| Teraspeed Modeling Services.
| http://www.teraspeed.com
[IBIS Ver]   4.0
[Comment Char] |_char
[File Name]   lpc812m101fdh20_ht.ibs
[File Rev]   3.0
[Source]  Measured and created by Teraspeed Consulting Group LLC
[Date]   08-09-2013
[Notes]   Quality Check of this IBIS model: Model Passes IBIS Check
   Model parses into ICX IS. Simulation done with Hyperlynx.
   1. MIN TYP MAX information is based on Temperature and Voltage
   characteristics only.
   2. Package data measured using Tektronix IConnect Software.
   3. This model higher temperature range:  -40 to +105
[Disclaimer]
| Use: Teraspeed Consulting Group LLC ("Teraspeed") has
| licensed IBIS models to specific integrated circuit
| suppliers ("IC Vendors") for use and distribustion as
| follows: Each IC Vendor may use IBIS Models, and distribute
| them to IC Vendor's custumers to use solely for developing
| printed circute board designs. Users of this model may
| modify the IBIS model to suit its specific applications but
| rights to derivative works and such modifications shall belong
| to Teraspeed. No other distribution of these materials is
| permitted.
| DISCLAIMER OF WARRANTY: UNLESS OTHERWISE AGREED TO IN WRITING
| TERASPEED DISCLAIMS AND USER WAIVES ALL WARRANTIES, EXPRESS
| OR IMPLIED, INCLUDING WARRANTIES OF MERCHANTABILITY AND
| FITNESS FOR A PARTICULAR PURPOSE. IN NO EVENT SHALL
| TERASPEED BE LIABLE FOR ANY DIRECT OR INDIRECT DAMAGES,
| WHETHER IN CONTRACT OR TORT, INCLUDING, WITHOUT LIMITATION,
| LOST PROFITS, BUSINESS INTERRUPTION, OR LOST INFORMATION
| ARISING OUT OF THE USE OF OR THE INABILITY TO USE THE MODEL,
| EVEN IF TERASPEED HAS BEEN ADVISED OF THE POSSIBILITY OF SUCH
| DAMAGES.
[Copyright]
| This file is the legal property of Teraspeed Copyright(c) 2013.
| All other rights are reserved.
[Component] LPC812M101FDH20_HT
[Manufacturer] NXP Semiconductors
[Package]
| TSSOP20/SOT360-1
| variable   typ   min   max
R_pkg  1.000E-02  1.000E-02  1.000E-02
L_pkg  2.930E-09  2.280E-09  3.580E-09
C_pkg  8.810E-13  8.040E-13  9.580E-13
[Pin] signal_name  model_name  R_pin  L_pin C_pin
1   PIO0_17   pio0_17   1.000E-02   2.280E-09   8.040E-13
2   PIO0_13   pio0_13   1.000E-02   2.605E-09   8.425E-13
3   PIO0_12   pio0_12   1.000E-02   2.930E-09   8.810E-13
4   *RESET/PIO0_5   pio0_5   1.000E-02   3.255E-09   9.195E-13
5   PIO0_4/WAKEUP/*TRST   pio0_4   1.000E-02   3.580E-09   9.580E-13
6   SWCLK/PIO0_3/TCK   pio0_3   1.000E-02   3.580E-09   9.580E-13
7   SWDIO/PIO0_2/TMS   pio0_2   1.000E-02   3.255E-09   9.195E-13
8   PIO0_11   pio0_11   1.000E-02   2.930E-09   8.810E-13
9   PIO0_10   pio0_10   1.000E-02   2.605E-09   8.425E-13
10   PIO0_16   pio0_16   1.000E-02   2.280E-09   8.040E-13
11   PIO0_15   pio0_15   1.000E-02   2.280E-09   8.040E-13
12   PIO0_1/CMPI2/CLK/TDI   pio0_1   1.000E-02   2.605E-09   8.425E-13
13   PIO0_9/XTALOUT   pio0_9   1.000E-02   2.930E-09   8.810E-13
14   PIO0_8/XTALIN   pio0_8   1.000E-02   3.255E-09   9.195E-13
15   VDD   POWER   1.000E-02   3.580E-09   9.580E-13
16   VSS   GND   1.000E-02   3.580E-09   9.580E-13
17   PIO0_7   pio0_7   1.000E-02   3.255E-09   9.195E-13
18   PIO0_6/VDDCMP   pio0_6   1.000E-02   2.930E-09   8.810E-13
19   PIO0_0/CMPI1/TDO   pio0_0   1.000E-02   2.605E-09   8.425E-13
20   PIO0_14   pio0_14   1.000E-02   2.280E-09   8.040E-13
|******Normal Drive I/O's******
[Model Selector]  pio0_4
input_1.8v   input,no int pd/pu,vdd=1.8v
input_2.5v   input,no int pd/pu,vdd=2.5v
input_3.3v   input,no int pd/pu,vdd=3.3v
pd_1.8v   input,int pd,vdd=1.8v
pd_2.5v   input,int pd,vdd=2.5v
pd_3.3v   input,int pd,vdd=3.3v
pu_1.8v   input,int pu,vdd=1.8v | PWR-UP Default
pu_2.5v   input,int pu,vdd=2.5v | PWR-UP Default
pu_3.3v   input,int pu,vdd=3.3v | PWR-UP Default
io_1.8v   io,vdd=1.8v
io_2.5v   io,vdd=2.5v
io_3.3v   io,vdd=3.3v
io_odf_1.8v   fast open drain io,vdd=1.8v
io_odf_2.5v   fast open drain io,vdd=2.5v
io_odf_3.3v   fast open drain io,vdd=3.3v
[Model Selector]  pio0_5
input_1.8v   input,no int pd/pu,vdd=1.8v
input_2.5v   input,no int pd/pu,vdd=2.5v
input_3.3v   input,no int pd/pu,vdd=3.3v
pd_1.8v   input,int pd,vdd=1.8v
pd_2.5v   input,int pd,vdd=2.5v
pd_3.3v   input,int pd,vdd=3.3v
pu_1.8v   input,int pu,vdd=1.8v | PWR-UP/Reset Default
pu_2.5v   input,int pu,vdd=2.5v | PWR-UP/Reset Default
pu_3.3v   input,int pu,vdd=3.3v | PWR-UP/Reset Default
io_1.8v   io,vdd=1.8v
io_2.5v   io,vdd=2.5v
io_3.3v   io,vdd=3.3v
io_odf_1.8v   fast open drain io,vdd=1.8v
io_odf_2.5v   fast open drain io,vdd=2.5v
io_odf_3.3v   fast open drain io,vdd=3.3v
[Model Selector]  pio0_6
input_1.8v   input,no int pd/pu,vdd=1.8v
input_2.5v   input,no int pd/pu,vdd=2.5v
input_3.3v   input,no int pd/pu,vdd=3.3v
pd_1.8v   input,int pd,vdd=1.8v
pd_2.5v   input,int pd,vdd=2.5v
pd_3.3v   input,int pd,vdd=3.3v
pu_1.8v   input,int pu,vdd=1.8v | PWR-UP/Reset Default
pu_2.5v   input,int pu,vdd=2.5v | PWR-UP/Reset Default
pu_3.3v   input,int pu,vdd=3.3v | PWR-UP/Reset Default
io_1.8v   io,vdd=1.8v
io_2.5v   io,vdd=2.5v
io_3.3v   io,vdd=3.3v
io_odf_1.8v   fast open drain io,vdd=1.8v
io_odf_2.5v   fast open drain io,vdd=2.5v
io_odf_3.3v   fast open drain io,vdd=3.3v
[Model Selector]  pio0_14
input_1.8v   input,no int pd/pu,vdd=1.8v
input_2.5v   input,no int pd/pu,vdd=2.5v
input_3.3v   input,no int pd/pu,vdd=3.3v
pd_1.8v   input,int pd,vdd=1.8v
pd_2.5v   input,int pd,vdd=2.5v
pd_3.3v   input,int pd,vdd=3.3v
pu_1.8v   input,int pu,vdd=1.8v | PWR-UP/Reset Default
pu_2.5v   input,int pu,vdd=2.5v | PWR-UP/Reset Default
pu_3.3v   input,int pu,vdd=3.3v | PWR-UP/Reset Default
io_1.8v   io,vdd=1.8v
io_2.5v   io,vdd=2.5v
io_3.3v   io,vdd=3.3v
io_odf_1.8v   fast open drain io,vdd=1.8v
io_odf_2.5v   fast open drain io,vdd=2.5v
io_odf_3.3v   fast open drain io,vdd=3.3v
[Model Selector]  pio0_15
input_1.8v   input,no int pd/pu,vdd=1.8v
input_2.5v   input,no int pd/pu,vdd=2.5v
input_3.3v   input,no int pd/pu,vdd=3.3v
pd_1.8v   input,int pd,vdd=1.8v
pd_2.5v   input,int pd,vdd=2.5v
pd_3.3v   input,int pd,vdd=3.3v
pu_1.8v   input,int pu,vdd=1.8v | PWR-UP/Reset Default
pu_2.5v   input,int pu,vdd=2.5v | PWR-UP/Reset Default
pu_3.3v   input,int pu,vdd=3.3v | PWR-UP/Reset Default
io_1.8v   io,vdd=1.8v
io_2.5v   io,vdd=2.5v
io_3.3v   io,vdd=3.3v
io_odf_1.8v   fast open drain io,vdd=1.8v
io_odf_2.5v   fast open drain io,vdd=2.5v
io_odf_3.3v   fast open drain io,vdd=3.3v
[Model Selector]  pio0_16
input_1.8v   input,no int pd/pu,vdd=1.8v
input_2.5v   input,no int pd/pu,vdd=2.5v
input_3.3v   input,no int pd/pu,vdd=3.3v
pd_1.8v   input,int pd,vdd=1.8v
pd_2.5v   input,int pd,vdd=2.5v
pd_3.3v   input,int pd,vdd=3.3v
pu_1.8v   input,int pu,vdd=1.8v | PWR-UP/Reset Default
pu_2.5v   input,int pu,vdd=2.5v | PWR-UP/Reset Default
pu_3.3v   input,int pu,vdd=3.3v | PWR-UP/Reset Default
io_1.8v   io,vdd=1.8v
io_2.5v   io,vdd=2.5v
io_3.3v   io,vdd=3.3v
io_odf_1.8v   fast open drain io,vdd=1.8v
io_odf_2.5v   fast open drain io,vdd=2.5v
io_odf_3.3v   fast open drain io,vdd=3.3v
[Model Selector]  pio0_17
input_1.8v   input,no int pd/pu,vdd=1.8v
input_2.5v   input,no int pd/pu,vdd=2.5v
input_3.3v   input,no int pd/pu,vdd=3.3v
pd_1.8v   input,int pd,vdd=1.8v
pd_2.5v   input,int pd,vdd=2.5v
pd_3.3v   input,int pd,vdd=3.3v
pu_1.8v   input,int pu,vdd=1.8v | PWR-UP/Reset Default
pu_2.5v   input,int pu,vdd=2.5v | PWR-UP/Reset Default
pu_3.3v   input,int pu,vdd=3.3v | PWR-UP/Reset Default
io_1.8v   io,vdd=1.8v
io_2.5v   io,vdd=2.5v
io_3.3v   io,vdd=3.3v
io_odf_1.8v   fast open drain io,vdd=1.8v
io_odf_2.5v   fast open drain io,vdd=2.5v
io_odf_3.3v   fast open drain io,vdd=3.3v
|******Normal Drive I/O's w/Analog Func ******
[Model Selector]  pio0_0
input_1.8v   input,no int pd/pu,vdd=1.8v
input_2.5v   input,no int pd/pu,vdd=2.5v
input_3.3v   input,no int pd/pu,vdd=3.3v
pd_1.8v   input,int pd,vdd=1.8v
pd_2.5v   input,int pd,vdd=2.5v
pd_3.3v   input,int pd,vdd=3.3v
pu_1.8v   input,int pu,vdd=1.8v | PWR-UP/Reset Default
pu_2.5v   input,int pu,vdd=2.5v | PWR-UP/Reset Default
pu_3.3v   input,int pu,vdd=3.3v | PWR-UP/Reset Default
io_1.8v   io,vdd=1.8v
io_2.5v   io,vdd=2.5v
io_3.3v   io,vdd=3.3v
io_odf_1.8v   fast open drain io,vdd=1.8v
io_odf_2.5v   fast open drain io,vdd=2.5v
io_odf_3.3v   fast open drain io,vdd=3.3v
term   analog comparator input1
[Model Selector]  pio0_1
input_1.8v   input,no int pd/pu,vdd=1.8v
input_2.5v   input,no int pd/pu,vdd=2.5v
input_3.3v   input,no int pd/pu,vdd=3.3v
pd_1.8v   input,int pd,vdd=1.8v
pd_2.5v   input,int pd,vdd=2.5v
pd_3.3v   input,int pd,vdd=3.3v
pu_1.8v   input,int pu,vdd=1.8v | PWR-UP/Reset Default
pu_2.5v   input,int pu,vdd=2.5v | PWR-UP/Reset Default
pu_3.3v   input,int pu,vdd=3.3v | PWR-UP/Reset Default
io_1.8v   io,vdd=1.8v
io_2.5v   io,vdd=2.5v
io_3.3v   io,vdd=3.3v
io_odf_1.8v   fast open drain io,vdd=1.8v
io_odf_2.5v   fast open drain io,vdd=2.5v
io_odf_3.3v   fast open drain io,vdd=3.3v
term   analog comparator input2
[Model Selector]  pio0_8
input_1.8v   input,no int pd/pu,vdd=1.8v
input_2.5v   input,no int pd/pu,vdd=2.5v
input_3.3v   input,no int pd/pu,vdd=3.3v
pd_1.8v   input,int pd,vdd=1.8v
pd_2.5v   input,int pd,vdd=2.5v
pd_3.3v   input,int pd,vdd=3.3v
pu_1.8v   input,int pu,vdd=1.8v | PWR-UP/Reset Default
pu_2.5v   input,int pu,vdd=2.5v | PWR-UP/Reset Default
pu_3.3v   input,int pu,vdd=3.3v | PWR-UP/Reset Default
io_1.8v   io,vdd=1.8v
io_2.5v   io,vdd=2.5v
io_3.3v   io,vdd=3.3v
io_odf_1.8v   fast open drain io,vdd=1.8v
io_odf_2.5v   fast open drain io,vdd=2.5v
io_odf_3.3v   fast open drain io,vdd=3.3v
term   analog xtal in
[Model Selector]  pio0_9
input_1.8v   input,no int pd/pu,vdd=1.8v
input_2.5v   input,no int pd/pu,vdd=2.5v
input_3.3v   input,no int pd/pu,vdd=3.3v
pd_1.8v   input,int pd,vdd=1.8v
pd_2.5v   input,int pd,vdd=2.5v
pd_3.3v   input,int pd,vdd=3.3v
pu_1.8v   input,int pu,vdd=1.8v | PWR-UP/Reset Default
pu_2.5v   input,int pu,vdd=2.5v | PWR-UP/Reset Default
pu_3.3v   input,int pu,vdd=3.3v | PWR-UP/Reset Default
io_1.8v   io,vdd=1.8v
io_2.5v   io,vdd=2.5v
io_3.3v   io,vdd=3.3v
io_odf_1.8v   fast open drain io,vdd=1.8v
io_odf_2.5v   fast open drain io,vdd=2.5v
io_odf_3.3v   fast open drain io,vdd=3.3v
term   analog xtal out
|******High Drive(source) I/O's******
[Model Selector]  pio0_2
input_1.8v   input,no int pd/pu,vdd=1.8v
input_2.5v   input,no int pd/pu,vdd=2.5v
input_3.3v   input,no int pd/pu,vdd=3.3v
pd_1.8v   input,int pd,vdd=1.8v
pd_2.5v   input,int pd,vdd=2.5v
pd_3.3v   input,int pd,vdd=3.3v
pu_1.8v   input,int pu,vdd=1.8v | PWR-UP/Reset Default
pu_2.5v   input,int pu,vdd=2.5v | PWR-UP/Reset Default
pu_3.3v   input,int pu,vdd=3.3v | PWR-UP/Reset Default
hi_drv_io_1.8v  io,hi src drv,vdd=1.8v
hi_drv_io_2.5v  io,hi src drv,vdd=2.5v
hi_drv_io_3.3v  io,hi src drv,vdd=3.3v
io_ods_1.8v   slow open drain io,vdd=1.8v
io_ods_2.5v   slow open drain io,vdd=2.5v
io_ods_3.3v   slow open drain io,vdd=3.3v
[Model Selector]  pio0_3
input_1.8v   input,no int pd/pu,vdd=1.8v
input_2.5v   input,no int pd/pu,vdd=2.5v
input_3.3v   input,no int pd/pu,vdd=3.3v
pd_1.8v   input,int pd,vdd=1.8v
pd_2.5v   input,int pd,vdd=2.5v
pd_3.3v   input,int pd,vdd=3.3v
pu_1.8v   input,int pu,vdd=1.8v | PWR-UP/Reset Default
pu_2.5v   input,int pu,vdd=2.5v | PWR-UP/Reset Default
pu_3.3v   input,int pu,vdd=3.3v | PWR-UP/Reset Default
hi_drv_io_1.8v  io,hi src drv,vdd=1.8v
hi_drv_io_2.5v  io,hi src drv,vdd=2.5v
hi_drv_io_3.3v  io,hi src drv,vdd=3.3v
io_ods_1.8v   slow open drain io,vdd=1.8v
io_ods_2.5v   slow open drain io,vdd=2.5v
io_ods_3.3v   slow open drain io,vdd=3.3v
[Model Selector]  pio0_7
input_1.8v   input,no int pd/pu,vdd=1.8v
input_2.5v   input,no int pd/pu,vdd=2.5v
input_3.3v   input,no int pd/pu,vdd=3.3v
pd_1.8v   input,int pd,vdd=1.8v
pd_2.5v   input,int pd,vdd=2.5v
pd_3.3v   input,int pd,vdd=3.3v
pu_1.8v   input,int pu,vdd=1.8v | PWR-UP/Reset Default
pu_2.5v   input,int pu,vdd=2.5v | PWR-UP/Reset Default
pu_3.3v   input,int pu,vdd=3.3v | PWR-UP/Reset Default
hi_drv_io_1.8v  io,hi src drv,vdd=1.8v
hi_drv_io_2.5v  io,hi src drv,vdd=2.5v
hi_drv_io_3.3v  io,hi src drv,vdd=3.3v
io_ods_1.8v   slow open drain io,vdd=1.8v
io_ods_2.5v   slow open drain io,vdd=2.5v
io_ods_3.3v   slow open drain io,vdd=3.3v
[Model Selector]  pio0_12
input_1.8v   input,no int pd/pu,vdd=1.8v
input_2.5v   input,no int pd/pu,vdd=2.5v
input_3.3v   input,no int pd/pu,vdd=3.3v
pd_1.8v   input,int pd,vdd=1.8v
pd_2.5v   input,int pd,vdd=2.5v
pd_3.3v   input,int pd,vdd=3.3v
pu_1.8v   input,int pu,vdd=1.8v | PWR-UP/Reset Default
pu_2.5v   input,int pu,vdd=2.5v | PWR-UP/Reset Default
pu_3.3v   input,int pu,vdd=3.3v | PWR-UP/Reset Default
hi_drv_io_1.8v  io,hi src drv,vdd=1.8v
hi_drv_io_2.5v  io,hi src drv,vdd=2.5v
hi_drv_io_3.3v  io,hi src drv,vdd=3.3v
io_ods_1.8v   slow open drain io,vdd=1.8v
io_ods_2.5v   slow open drain io,vdd=2.5v
io_ods_3.3v   slow open drain io,vdd=3.3v
[Model Selector]  pio0_13
input_1.8v   input,no int pd/pu,vdd=1.8v
input_2.5v   input,no int pd/pu,vdd=2.5v
input_3.3v   input,no int pd/pu,vdd=3.3v
pd_1.8v   input,int pd,vdd=1.8v
pd_2.5v   input,int pd,vdd=2.5v
pd_3.3v   input,int pd,vdd=3.3v
pu_1.8v   input,int pu,vdd=1.8v | PWR-UP/Reset Default
pu_2.5v   input,int pu,vdd=2.5v | PWR-UP/Reset Default
pu_3.3v   input,int pu,vdd=3.3v | PWR-UP/Reset Default
hi_drv_io_1.8v  io,hi src drv,vdd=1.8v
hi_drv_io_2.5v  io,hi src drv,vdd=2.5v
hi_drv_io_3.3v  io,hi src drv,vdd=3.3v
io_ods_1.8v   slow open drain io,vdd=1.8v
io_ods_2.5v   slow open drain io,vdd=2.5v
io_ods_3.3v   slow open drain io,vdd=3.3v
|******Dedicated Open Drain I/O's******
[Model Selector]  pio0_10
i2c_io_1.8v   i2c true open drain io,vdd=1.8v
i2c_io_2.5v   i2c true open drain io,vdd=2.5v
i2c_io_3.3v   i2c true open drain io,vdd=3.3v
[Model Selector]  pio0_11
i2c_io_1.8v   i2c true open drain io,vdd=1.8v
i2c_io_2.5v   i2c true open drain io,vdd=2.5v
i2c_io_3.3v   i2c true open drain io,vdd=3.3v
[Model] term
Model_type Terminator
C_comp  0pF 0pF 0pF
| variable typ   min   max
[Voltage Range]   3.30000V  3.00000V  3.60000V
[POWER Clamp Reference]  3.30000V  3.00000V  3.60000V
[GND Clamp Reference]   0.00000V  0.00000V  0.00000V
[Temperature Range]   25   105   -40
| Models and submodels in the file (25): input_1.8v (Input), input_2.5v (Input), input_3.3v (Input), pd_1.8v (Input), pd_2.5v (Input), pd_3.3v (Input), pu_1.8v (Input), pu_2.5v (Input), pu_3.3v (Input), hi_drv_io_1.8v (I/O), hi_drv_io_2.5v (I/O), hi_drv_io_3.3v (I/O), io_1.8v (I/O), io_2.5v (I/O), io_3.3v (I/O), i2c_io_1.8v (I/O_open_drain), i2c_io_2.5v (I/O_open_drain), i2c_io_3.3v (I/O_open_drain), io_odf_1.8v (I/O_open_drain), io_odf_2.5v (I/O_open_drain), io_odf_3.3v (I/O_open_drain), io_ods_1.8v (I/O_open_drain), io_ods_2.5v (I/O_open_drain), io_ods_3.3v (I/O_open_drain), term (Terminator)
